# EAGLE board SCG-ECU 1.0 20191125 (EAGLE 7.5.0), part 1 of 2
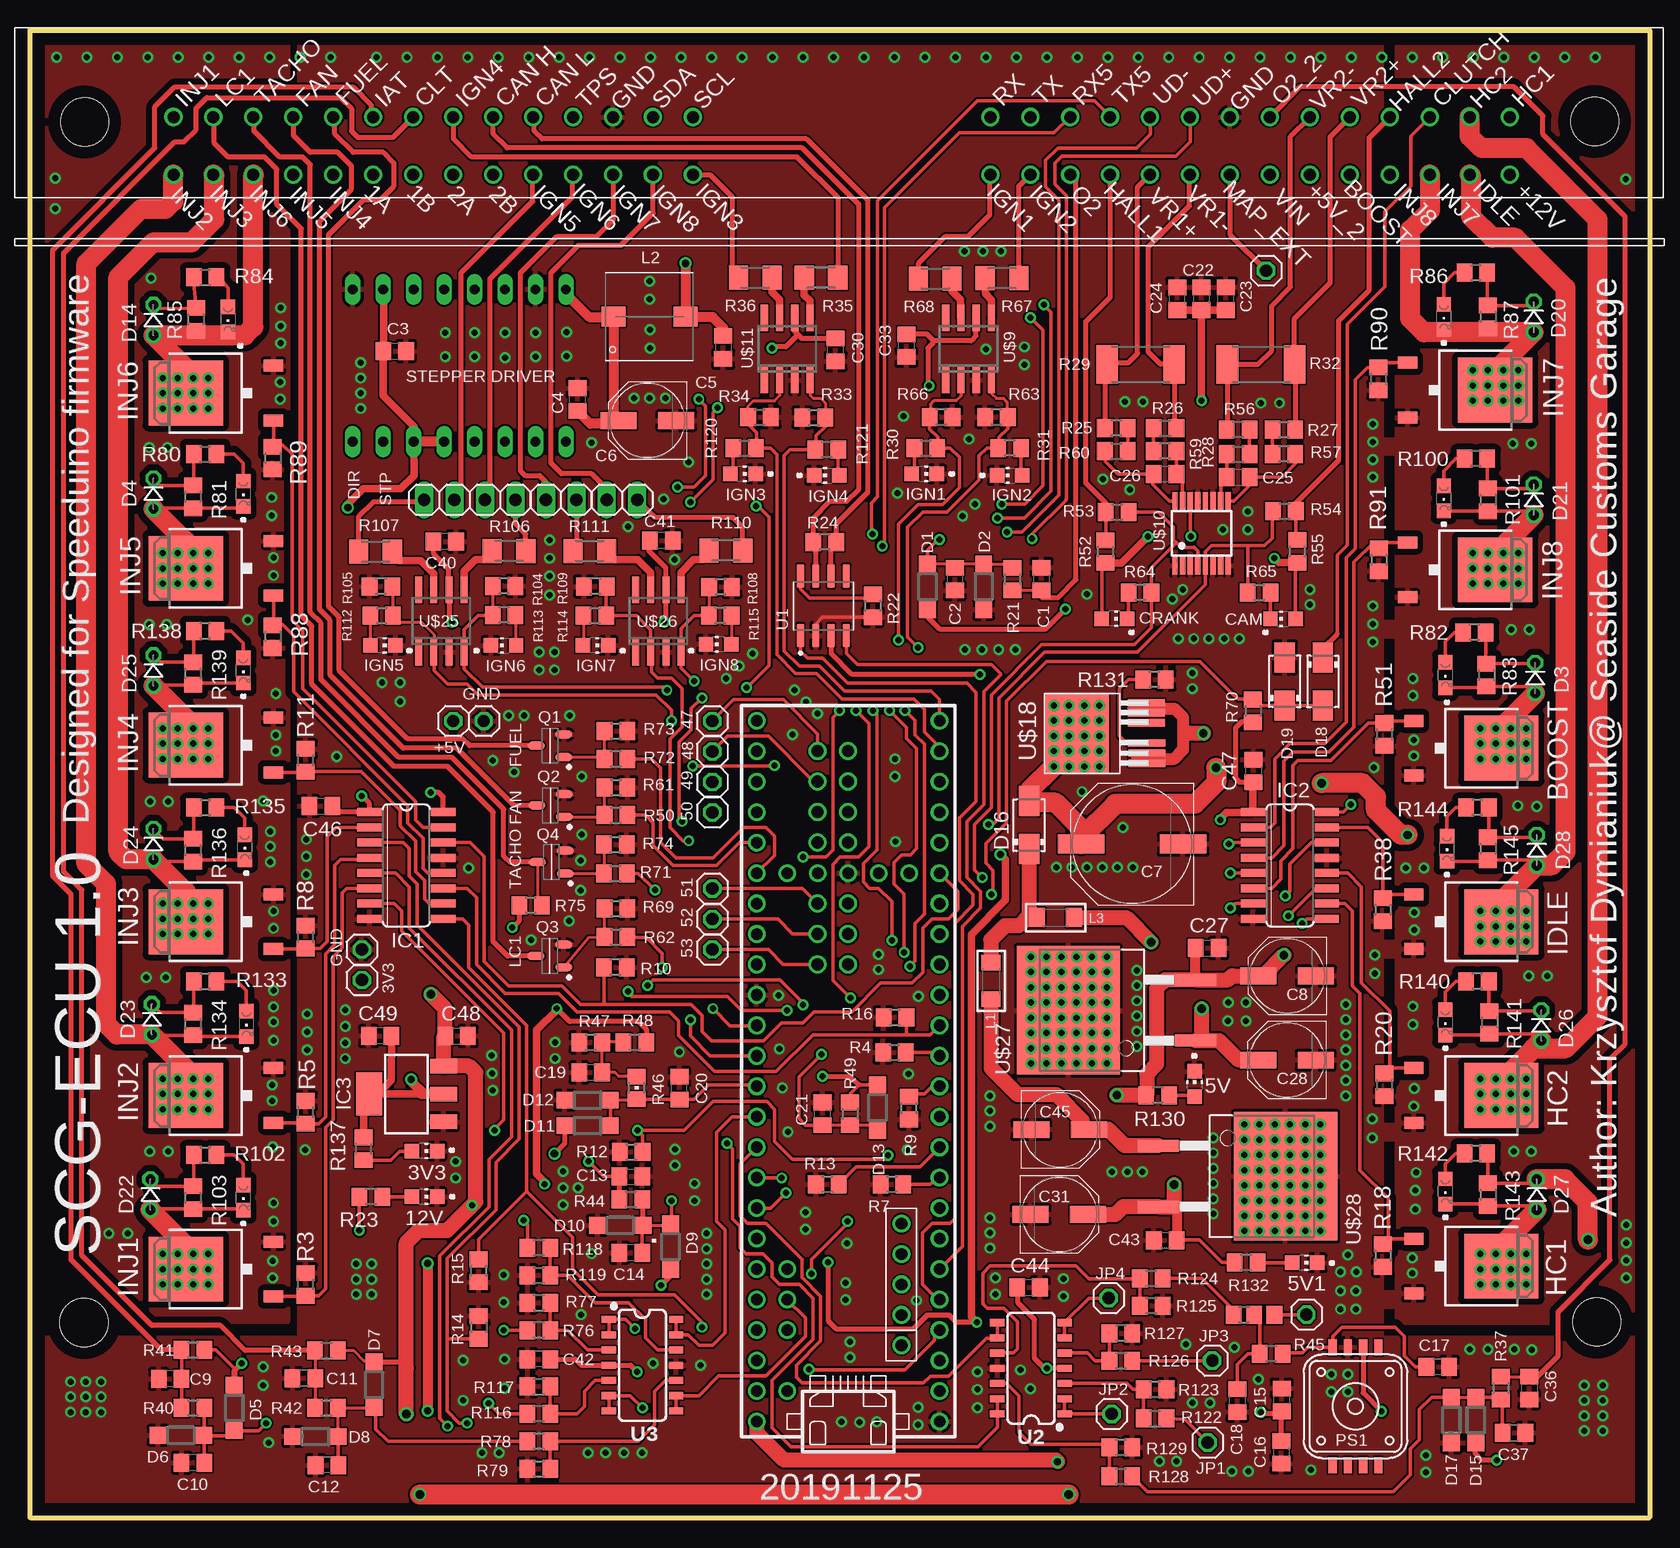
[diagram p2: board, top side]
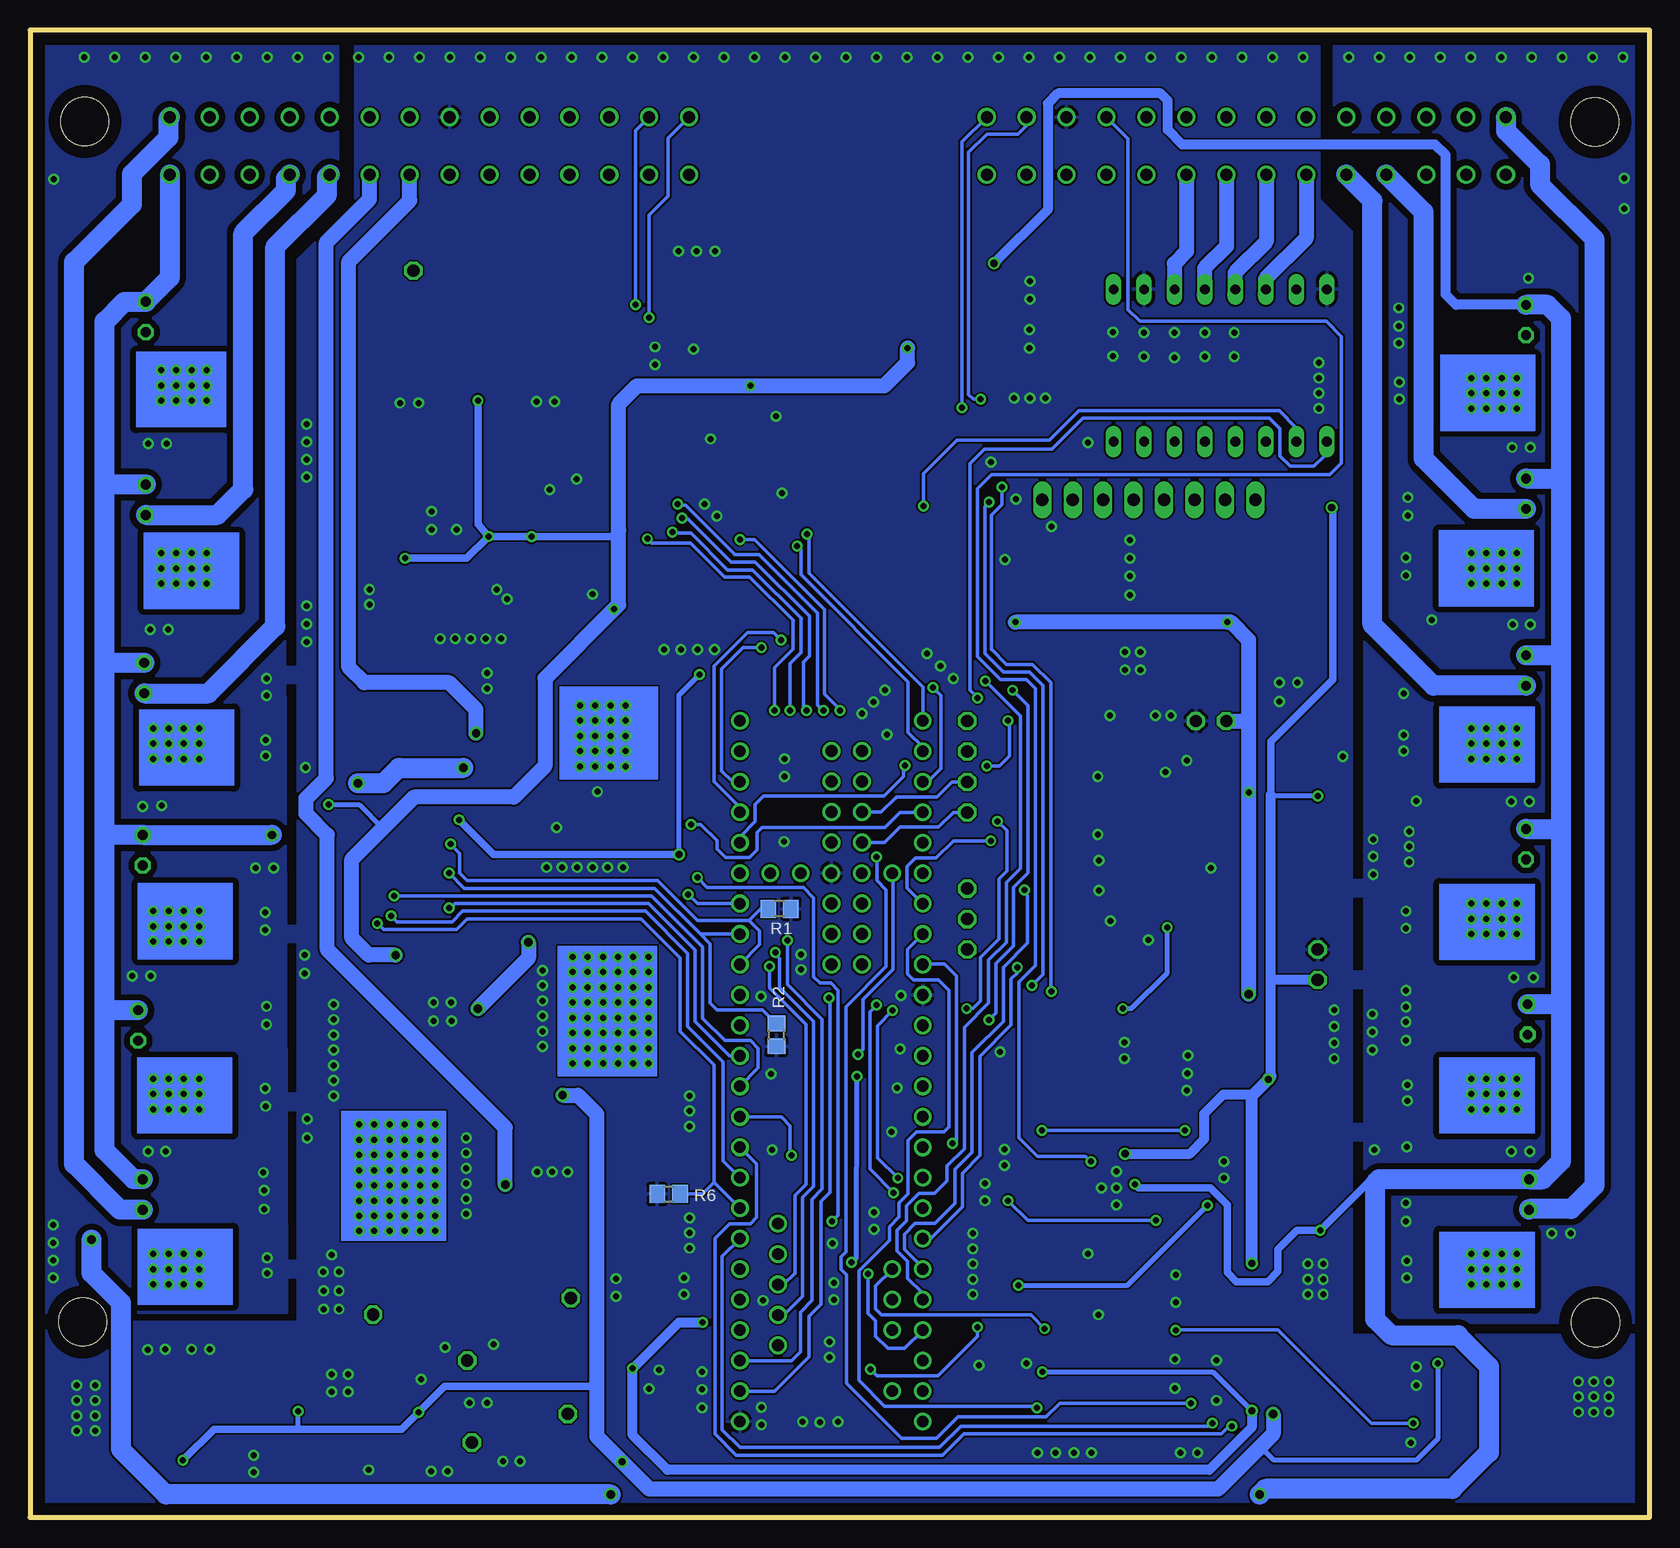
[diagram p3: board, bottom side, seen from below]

Size 135 x 124 mm. Coordinates in mm from the lower left corner, seen from the top.
Outline: 0,0 0,124 135,124 135,0 0,0
Copper layers (1*16): Top 0.035mm / dielectric 1.5mm / Bottom 0.035mm
Design rules "default *": minimum track width 10mil, minimum drill 24mil, track to track 6mil, track to pad 6mil, pad to pad 6mil, via to via 6mil, smd to smd 6mil, copper to edge 40mil, drill to drill 8mil, minimum pad ring 10mil, minimum via ring 8mil, stop-mask expansion 4mil, vias tented up to drill 20mil, thermal gap 10mil
Holes 4 mm at 4.5,16.25 130.61,16.31

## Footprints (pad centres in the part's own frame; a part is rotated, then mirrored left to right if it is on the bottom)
CHIP-LED0805 = smd 1.2 x 1.2: A 0,-1.05; C 0,1.05
C0805 = smd 1.3 x 1.5: 1 -0.95,0; 2 0.95,0
PANASONIC_D = smd 3 x 1.4: + 2.4,0; - -2.4,0
PANASONIC_G = smd 3.9 x 1.6: + 4.25,0; - -4.25,0
SOD123 = smd 1.4 x 1.4: A 1.9,0; C -1.9,0
D-2.5 = drill 0.813 octagon: A 1.27,0; C -1.27,0
DO214AC = smd 2.5 x 1.7: A 2,0; C -2,0
SO16 = smd 0.66 x 2.032: 1 -4.445,-3.073; 2 -3.175,-3.073; 3 -1.905,-3.073; 4 -0.635,-3.073; 5 0.635,-3.073; 6 1.905,-3.073; 7 3.175,-3.073; 8 4.445,-3.073; 9 4.445,3.073; 10 3.175,3.073; 11 1.905,3.073; 12 0.635,3.073; 13 -0.635,3.073; 14 -1.905,3.073; 15 -3.175,3.073; 16 -4.445,3.073
SOT223 = smd 1.219 x 2.235: 1 -2.311,-3.099; 2 0,-3.099; 3 2.311,-3.099 | smd 3.6 x 2.2: TAB 0,3.099
1X01 = drill 1.016 octagon: 1 0,0
1X02 = drill 1.016 long: 1 -1.27,0; 2 1.27,0
A0R-JMP = smd 1.5 x 1.3: 1 0,1.7; 2 0,0; 3 0,-1.7
L1206 = smd 1.3 x 1.6: 1 -1.524,0; 2 1.524,0
WE-PD_7332/7345_PLASTIC_BASE = smd 1.7 x 2: 1 0,3; 2 0,-3
CHIPLED_0805 = smd 1.2 x 1.2: A 0,-1.05; C 0,1.05
1317A = smd 1.346 x 0.686: 1 4.915,-1.905; 2 4.915,-0.635; 3 4.915,0.635; 4 4.915,1.905; 5 -4.915,1.905; 6 -4.915,0.635; 7 -4.915,-0.635; 8 -4.915,-1.905
SOT95P280X135-3N = smd 1.4 x 0.65: 1 -1.15,0.95; 2 -1.15,-0.95; 3 1.15,0
R0805 = smd 1.3 x 1.5: 1 -0.95,0; 2 0.95,0
R2512 = smd 1.8 x 3.2: 1 -2.8,0; 2 2.8,0
M1206 = smd 1.6 x 2: 1 -1.4,0; 2 1.4,0
STEP-STICK = drill 0.8 long: 1A -8.89,-7.62; 1B -8.89,-5.08; 2A -8.89,-2.54; 2B -8.89,0; DIR 3.81,-12.7; EN 3.81,5.08; GND -8.89,-12.7; GNDM -8.89,2.54; MS1 3.81,2.54; MS2 3.81,0; MS3 3.81,-2.54; RST 3.81,-5.08; SLP 3.81,-7.62; SPT 3.81,-10.16; VCC -8.89,-10.16; VMOT -8.89,5.08
SOIC127P600X175-8N = smd 1.97 x 0.6: 1 -2.475,1.905; 2 -2.475,0.635; 3 -2.475,-0.635; 4 -2.475,-1.905; 5 2.475,-1.905; 6 2.475,-0.635; 7 2.475,0.635; 8 2.475,1.905
SO14 = smd 0.6 x 1.2: 1 -3.175,-2.8; 2 -1.905,-2.8; 3 -0.635,-2.8; 4 0.635,-2.8; 5 1.905,-2.8; 6 3.175,-2.8; 7 4.445,-2.8; 8 4.445,2.8; 9 3.175,2.8; 10 1.905,2.8; 11 0.635,2.8; 12 -0.635,2.8; 13 -1.905,2.8; 14 -3.175,2.8
TEENSY_3.5/3.6 = drill 0.965: 0/RX -25.4,-7.62; 1/TX -22.86,-7.62; 2 -20.32,-7.62; 3/CANTX -17.78,-7.62; 3V3 7.62,-7.62; 3V3_2 17.78,-2.54; 3V3_LO -22.86,7.62; 4/CANRX -15.24,-7.62; 5 -12.7,-7.62; 6 -10.16,-7.62; 7 -7.62,-7.62; 8 -5.08,-7.62; 9/CS -2.54,-7.62; 10/CS 0,-7.62; 11/MOSI 2.54,-7.62; 12/MISO 5.08,-7.62; 13/SCK 5.08,7.62; 14/A0 2.54,7.62; 15/A1 0,7.62; 16/A2 -2.54,7.62; 17/A3 -5.08,7.62; 18/A4/SDA -7.62,7.62; 19/A5/SCL -10.16,7.62; 20/A6 -12.7,7.62; 21/A7 -15.24,7.62; 21/DAC0 12.7,7.62; 22/A8 -17.78,7.62; 23/A9 -20.32,7.62; 24 10.16,-7.62; 25 12.7,-7.62; 26 15.24,-7.62; 27 17.78,-7.62; 28 20.32,-7.62; 29 22.86,-7.62; 30 25.4,-7.62; 31/A12 27.94,-7.62; 32/A13 30.48,-7.62; 33/A14 30.48,7.62; 34/A15 27.94,7.62; 35/A16 25.4,7.62; 36/A17 22.86,7.62; 37/A18 20.32,7.62; 38/A19 17.78,7.62; 39/A20 15.24,7.62; A10 -17.78,5.08; A11 -15.24,5.08; A22/DAC1 10.16,7.62; AGND -25.4,7.62; AREF -20.32,5.08; GND -27.94,-7.62; GND2 7.62,7.62; GND3 17.78,0; PROG 17.78,2.54; RESET 17.78,5.08; U5V -21.59,-4.445; UD+ -16.51,-4.445; UD- -19.05,-4.445; UGND1 -13.97,-4.445; UGND2 -11.43,-4.445; VBAT 17.78,-5.08; VIN -27.94,7.62; VUSB -25.4,5.08 | drill 1: 40 10.16,0; 41 12.7,0; 42 15.24,0; 43 20.32,0; 44 22.86,0; 45 25.4,0; 46 27.94,0; 47 27.94,2.54; 48 25.4,2.54; 49 22.86,2.54; 50 20.32,2.54; 51 15.24,2.54; 52 12.7,2.54; 53 10.16,2.54
DPAK_N-CHANNEL_MOSFET = smd 5.4 x 6.2: D 0,1.23 | smd 1 x 1.6: G -2.28,-6.07; S 2.28,-6.07
SO-8 = smd 0.6 x 2.2: 1 -1.905,-2.6; 2 -0.635,-2.6; 3 0.635,-2.6; 4 1.905,-2.6; 5 1.905,2.6; 6 0.635,2.6; 7 -0.635,2.6; 8 -1.905,2.6
QSOP16 = smd 0.45 x 1.5: 1 -2.223,-2.69; 2 -1.587,-2.69; 3 -0.953,-2.69; 4 -0.318,-2.69; 5 0.318,-2.69; 6 0.953,-2.69; 7 1.587,-2.69; 8 2.223,-2.69; 9 2.223,2.69; 10 1.587,2.69; 11 0.953,2.69; 12 0.318,2.69; 13 -0.318,2.69; 14 -0.953,2.69; 15 -1.587,2.69; 16 -2.223,2.69
56PIN_CONNECTOR = drill 1: 1 -55.35,1.66; 2 -52.02,1.66; 3 -48.69,1.66; 4 -45.36,1.66; 5 -42.03,1.66; 6 -38.7,1.66; 7 -35.37,1.66; 8 -32.04,1.66; 9 -28.71,1.66; 10 -25.38,1.66; 11 -22.05,1.66; 12 -18.72,1.66; 13 -15.39,1.66; 14 -12.06,1.66; 15 -55.35,-3.14; 16 -52.02,-3.14; 17 -48.69,-3.14; 18 -45.36,-3.14; 19 -42.03,-3.14; 20 -38.7,-3.14; 21 -35.37,-3.14; 22 -32.04,-3.14; 23 -28.71,-3.14; 24 -25.38,-3.14; 25 -22.05,-3.14; 26 -18.72,-3.14; 27 -15.39,-3.14; 28 -12.06,-3.14; 29 12.74,1.66; 30 16.07,1.66; 31 19.4,1.66; 32 22.73,1.66; 33 26.06,1.66; 34 29.39,1.66; 35 32.72,1.66; 36 36.05,1.66; 37 39.38,1.66; 38 42.71,1.66; 39 46.04,1.66; 40 49.37,1.66; 41 52.7,1.66; 42 56.03,1.66; 43 12.74,-3.14; 44 16.07,-3.14; 45 19.4,-3.14; 46 22.73,-3.14; 47 26.06,-3.14; 48 29.39,-3.14; 49 32.72,-3.14; 50 36.05,-3.14; 51 39.38,-3.14; 52 42.71,-3.14; 53 46.04,-3.14; 54 49.37,-3.14; 55 52.7,-3.14; 56 56.03,-3.14 | hole 4: -62.76,1.24; 63.12,1.28
VN5R003H-E_HPAK_TO267_7 = smd 0.6 x 3.1: 1 -2.53,1.65; 2 -1.68,1.65; 3 -0.83,1.66; 5 0.85,1.67; 6 1.68,1.67; 7 2.53,1.67 | smd 6.5 x 5.3: 4 -0.05,7.45
TO263-3 = smd 1 x 3.4: 1 -2.54,-6.6; 3 2.54,-6.6 | smd 10.7 x 8.6: TAB 0,4

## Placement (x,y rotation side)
3V3  [CHIP-LED0805]  32.89,30.56 270 top
5V  [CHIP-LED0805]  97.08,36.14 0 top
5V1  [CHIP-LED0805]  106.25,21.23 270 top
12V  [CHIP-LED0805]  32.89,26.75 270 top
C1  100nF  [C0805]  84.33,78.23 90 top
C2  220nF  [C0805]  77.09,78.23 270 top
C3  100nF  [C0805]  30.4,97.23 0 top
C4  100nF 50V  [C0805]  45.64,93.19 90 top
C5  100nF 50V  [C0805]  57.78,97.54 270 top
C6  100uF 35V  [PANASONIC_D]  51.46,91.44 180 top
C7  470uF 50V  [PANASONIC_G]  91.87,56.13 180 top
C8  220uF  [PANASONIC_D]  104.8,45.14 180 top
C9  100nF  [C0805]  11.68,11.56 180 top
C10  220nF  [C0805]  13.59,4.57 180 top
C11  100nF  [C0805]  22.83,11.61 180 top
C12  220nF  [C0805]  24.77,4.37 180 top
C13  100nF  [C0805]  50.09,28.42 0 top
C14  220nF  [C0805]  50.09,22.07 180 top
C15  1uF  [C0805]  104.34,9.8 90 top
C16  100nF  [C0805]  104.29,5.44 270 top
C17  100nF  [C0805]  117.35,12.55 180 top
C18  220nF  [C0805]  100.63,9.75 90 top
C19  100nF  [C0805]  46.74,37.08 180 top
C20  220nF  [C0805]  54.13,35.79 90 top
C21  4.7nF  [C0805]  66.07,33.66 90 top
C22  10nF  [C0805]  97.66,101.6 90 top
C23  100nF  [C0805]  99.69,101.6 90 top
C24  1uF  [C0805]  95.63,101.6 90 top
C25  1nF  [C0805]  100.71,86.74 0 top
C26  1nF  [C0805]  94.61,86.99 0 top
C27  1uF  [C0805]  98.12,47.47 0 top
C28  220uF  [PANASONIC_D]  104.78,38.13 180 top
C30  1uF  [C0805]  67.16,97.33 90 top
C31  220uF  [PANASONIC_D]  85.8,25.27 0 top
C33  1uF  [C0805]  73.05,97.69 90 top
C36  100nF  [C0805]  124.97,10.79 270 top
C37  220nF  [C0805]  123.7,7.06 0 top
C40  1uF  [C0805]  34.57,81.36 180 top
C41  1uF  [C0805]  52.63,81.43 180 top
C42  100nF  [C0805]  42.42,13.21 180 top
C43  1uF  [C0805]  94.64,23.09 180 top
C44  100nF  [C0805]  83.24,19.18 0 top
C45  220uF  [PANASONIC_D]  85.88,32.33 0 top
C46  100nF  [C0805]  24.26,59.31 0 top
C47  100nF  [C0805]  101.98,62.23 270 top
C48  10uF  [C0805]  35.56,40.13 0 top
C49  10uF  [C0805]  29.18,40.13 180 top
D1  1N5819HW-7-F  [SOD123]  74.8,77.6 90 top
D2  1N5819HW-7-F  [SOD123]  79.5,77.6 270 top
D3  1N4001  [D-2.5]  125.48,69.98 270 top
D4  1N4001  [D-2.5]  10.29,85.34 270 top
D5  1N5819HW-7-F  [SOD123]  17.02,9.14 270 top
D6  1N5819HW-7-F  [SOD123]  12.57,6.86 180 top
D7  1N5819HW-7-F  [SOD123]  28.68,11.07 270 top
D8  1N5819HW-7-F  [SOD123]  23.8,6.76 180 top
D9  1N5819HW-7-F  [SOD123]  53.39,22.58 90 top
D10  1N5819HW-7-F  [SOD123]  49.2,24.36 180 top
D11  1N5819  [SOD123]  46.48,32.66 0 top
D12  1N5819  [SOD123]  46.48,34.8 180 top
D13  1N5819HW-7-F  [SOD123]  70.64,34.16 270 top
D14  1N4001  [D-2.5]  10.29,99.82 270 top
D15  1N5819HW-7-F  [SOD123]  120.52,8.13 90 top
D16  B340A 3A  [DO214AC]  83.29,57.71 90 top
D17  1N5819HW-7-F  [SOD123]  118.49,8.13 270 top
D18  1N4001 SMA  [DO214AC]  107.77,69.7 270 top
D19  1N4001 SMA  [DO214AC]  104.6,69.7 90 top
D20  1N4001  [D-2.5]  125.35,100.08 270 top
D21  1N4001  [D-2.5]  125.35,84.84 270 top
D22  1N4001  [D-2.5]  10.03,26.92 270 top
D23  1N4001  [D-2.5]  10.16,41.53 270 top
D24  1N4001  [D-2.5]  10.29,56.13 270 top
D25  1N4001  [D-2.5]  10.29,70.61 270 top
D26  1N4001  [D-2.5]  125.98,41.02 270 top
D27  1N4001  [D-2.5]  125.6,26.92 270 top
D28  1N4001  [D-2.5]  125.6,55.63 270 top
IC1  4504D  [SO16]  31.37,54.36 270 top
IC2  4504D  [SO16]  105.03,54.36 270 top
IC3  LM1117IMPX-3.3  [SOT223]  31.37,35.31 90 top
JP1  [1X01]  98.17,6.25 0 top
JP2  [1X01]  90.17,8.64 0 top
JP3  [1X01]  98.55,13.08 0 top
JP4  [1X01]  89.92,18.29 0 top
JP5  [1X01]  56.87,47.35 0 top
JP6  [1X01]  56.87,49.89 0 top
JP7  [1X01]  56.87,52.43 0 top
JP8  [1X01]  56.87,58.78 0 top
JP9  [1X01]  56.87,61.32 0 top
JP10  [1X01]  56.87,63.86 0 top
JP11  [1X01]  56.87,66.4 0 top
JP12  [1X01]  27.66,47.35 0 top
JP13  [1X01]  35.28,66.4 0 top
JP14  [1X01]  27.66,44.81 0 top
JP15  [1X02]  34.11,84.84 0 top
JP16  [1X02]  44.27,84.84 180 top
JP17  [1X02]  49.35,84.84 0 top
JP18  [1X02]  39.19,84.84 0 top
JP19  [1X01]  37.82,66.4 0 top
JP20  0R-JUMPA  [A0R-JMP]  102.03,16.92 90 top
JP21  [1X01]  106.4,16.92 0 top
JP22  [1X01]  103.05,103.94 0 top
L1  600R 2A  [L1206]  80.11,44.73 90 top
L2  8.2uH 2.7A  [WE-PD_7332/7345_PLASTIC_BASE]  51.64,100.1 90 top
L3  600R 2A  [L1206]  85.5,50.01 180 top
LED1  [CHIP-LED0805]  74.55,86.99 270 top
LED2  [CHIP-LED0805]  81.66,86.87 90 top
LED3  [CHIP-LED0805]  59.44,86.99 270 top
LED4  [CHIP-LED0805]  66.42,86.87 90 top
LED5  [CHIPLED_0805]  117.98,70.23 180 top
LED6  [CHIP-LED0805]  90.4,74.93 270 top
LED7  [CHIP-LED0805]  104.44,74.9 90 top
LED8  [CHIPLED_0805]  17.78,85.34 180 top
LED9  [CHIPLED_0805]  16.51,99.87 180 top
LED10  [CHIPLED_0805]  117.86,100.08 180 top
LED11  [CHIPLED_0805]  117.86,84.96 180 top
LED12  [CHIPLED_0805]  17.78,26.67 180 top
LED13  [CHIPLED_0805]  18.03,41.15 180 top
LED14  [CHIPLED_0805]  17.91,55.88 180 top
LED15  [CHIPLED_0805]  17.78,70.61 180 top
LED16  [CHIPLED_0805]  117.98,41.28 180 top
LED17  [CHIPLED_0805]  117.98,27.18 180 top
LED18  [CHIPLED_0805]  118.11,55.75 180 top
LED20  [CHIP-LED0805]  29.41,72.69 270 top
LED21  [CHIP-LED0805]  39.47,72.69 90 top
LED22  [CHIP-LED0805]  47.14,72.69 270 top
LED23  [CHIP-LED0805]  57.4,72.8 90 top
PS1  MPXH6400AC6T1  [1317A]  110.49,9.27 90 top
Q1  IRLML0030TRPBF  [SOT95P280X135-3N]  43.36,64.34 180 top
Q2  IRLML0030TRPBF  [SOT95P280X135-3N]  43.38,59.36 180 top
Q3  IRLML0030TRPBF  [SOT95P280X135-3N]  43.33,46.81 180 top
Q4  IRLML0030TRPBF  [SOT95P280X135-3N]  43.46,54.64 180 top
R1  10K  [R0805]  72.52,50.75 180 bottom
R2  10K  [R0805]  72.77,40.23 90 bottom
R3  68K  [R0805]  22.99,19.43 90 top
R4  10K  [R0805]  72.06,38.76 0 top
R5  68K  [R0805]  22.99,33.78 90 top
R6  10K  [R0805]  81.76,26.97 0 bottom
R7  10K  [R0805]  71.86,27.79 0 top
R8  68K  [R0805]  22.99,48.39 90 top
R9  10K  [R0805]  73.28,34.14 90 top
R10  10K  [R0805]  48.79,45.87 180 top
R11  68K  [R0805]  22.99,63.12 90 top
R12  10K  [R0805]  50.11,30.48 0 top
R13  10K  [R0805]  66.47,27.79 0 top
R14  10K  [R0805]  37.41,15.85 270 top
R15  10K  [R0805]  37.41,20.57 90 top
R16  10K  [R0805]  72.11,41.71 0 top
R18  68K  [R0805]  112.78,21.84 270 top
R20  68K  [R0805]  112.9,36.07 270 top
R21  470R  [R0805]  81.92,78.23 90 top
R22  10K  [R0805]  70.26,76 270 top
R23  2K7  [R0805]  28.42,26.75 180 top
R24  120R  [R0805]  66.24,81.31 180 top
R25  5K  [R0805]  90.55,90.8 180 top
R26  5K  [R0805]  94.61,90.8 0 top
R27  5K  [R0805]  104.52,90.68 0 top
R28  5K  [R0805]  100.71,88.65 0 top
R29  4K7 3W  [R2512]  92.58,96.14 0 top
R30  470R  [R0805]  74.68,89.15 0 top
R31  470R  [R0805]  81.66,89.15 180 top
R32  4K7 3W  [R2512]  102.62,96.14 0 top
R33  100K  [R0805]  65.33,91.69 0 top
R34  100K  [R0805]  60.81,91.72 0 top
R35  22R  [M1206]  65.94,103.35 0 top
R36  22R  [M1206]  60.45,103.35 180 top
R37  470R  [R0805]  122.61,10.79 270 top
R38  68K  [R0805]  112.78,50.67 270 top
R40  470R  [R0805]  13.59,9.14 0 top
R41  2K49  [R0805]  13.59,13.97 0 top
R42  470R  [R0805]  24.71,9.14 0 top
R43  2K49  [R0805]  24.71,13.92 0 top
R44  470R  [R0805]  50.09,26.52 0 top
R45  470R  [R0805]  103.45,13.64 180 top
R46  470R  [R0805]  50.55,35.81 270 top
R47  1K  [R0805]  46.74,39.62 0 top
R48  3K9  [R0805]  50.42,39.62 0 top
R49  1K  [R0805]  68.35,33.66 270 top
R50  100R  [R0805]  48.84,58.55 0 top
R51  68K  [R0805]  112.9,65.28 270 top
R52  10K  [R0805]  89.66,80.52 90 top
R53  1K  [R0805]  90.63,83.82 0 top
R54  1K  [R0805]  104.57,83.9 0 top
R55  10K  [R0805]  105.64,80.54 90 top
R56  5K  [R0805]  100.71,90.68 180 top
R57  5K  [R0805]  104.52,88.65 180 top
R59  5K  [R0805]  94.61,88.9 180 top
R60  5K  [R0805]  90.55,88.9 0 top
R61  47K  [R0805]  48.84,60.86 0 top
R62  100R  [R0805]  48.84,48.39 0 top
R63  100K  [R0805]  80.57,91.74 0 top
R64  10K  [R0805]  92.53,77.11 180 top
R65  10K  [R0805]  102.46,77.11 0 top
R66  100K  [R0805]  75.95,91.74 0 top
R67  22R  [M1206]  81.03,103.3 0 top
R68  22R  [M1206]  75.46,103.28 180 top
R69  47K  [R0805]  48.84,50.77 0 top
R70  2,2K  [R0805]  101.96,67.23 270 top
R71  100R  [R0805]  48.79,53.7 0 top
R72  100R  [R0805]  48.84,63.25 0 top
R73  47K  [R0805]  48.84,65.56 0 top
R74  47K  [R0805]  48.79,56.11 0 top
R75  10K  [R0805]  41.73,51.03 180 top
R76  180K +/-0.1%  [R0805]  42.42,15.62 180 top
R77  330K +/-0.1%  [R0805]  42.42,17.91 0 top
R78  180K +/-0.1%  [R0805]  42.42,6.35 180 top
R79  330K +/-0.1%  [R0805]  42.42,4.06 0 top
R80  2K7  [R0805]  14.61,88.65 0 top
R81  1K  [R0805]  13.59,85.09 270 top
R82  2K7  [R0805]  120.4,73.79 180 top
R83  1K  [R0805]  121.41,70.23 270 top
R84  2K7  [R0805]  14.61,103.38 0 top
R85  1K  [R0805]  13.84,99.87 270 top
R86  2K7  [R0805]  120.52,103.76 180 top
R87  1K  [R0805]  121.54,100.08 270 top
R88  68K  [R0805]  20.24,73.43 270 top
R89  68K  [R0805]  20.24,88.32 270 top
R90  68K  [R0805]  112.39,94.92 270 top
R91  68K  [R0805]  112.45,79.83 270 top
R100  2K7  [R0805]  120.52,88.27 180 top
R101  1K  [R0805]  121.54,84.84 270 top
R102  2K7  [R0805]  14.61,30.23 0 top
R103  1K  [R0805]  13.59,26.67 270 top
R104  100K  [R0805]  39.52,77.65 180 top
R105  100K  [R0805]  29.26,77.62 180 top
R106  22R  [M1206]  39.93,80.57 0 top
R107  22R  [M1206]  28.8,80.52 180 top
R108  100K  [R0805]  57.56,77.57 180 top
R109  100K  [R0805]  47.12,77.62 180 top
R110  22R  [M1206]  58.01,80.62 0 top
R111  22R  [M1206]  46.66,80.57 180 top
R112  470R  [R0805]  29.31,75.18 0 top
R113  470R  [R0805]  39.52,75.23 180 top
R114  470R  [R0805]  47.09,75.18 0 top
R115  470R  [R0805]  57.53,75.18 180 top
R116  180K +/-0.1%  [R0805]  42.42,8.64 180 top
R117  330K +/-0.1%  [R0805]  42.42,10.92 0 top
R118  180K +/-0.1%  [R0805]  42.42,22.48 180 top
R119  330K +/-0.1%  [R0805]  42.42,20.19 0 top
R120  470R  [R0805]  59.56,89.15 0 top
R121  470R  [R0805]  66.42,89.03 180 top
R122  180K +/-0.1%  [R0805]  93.78,8.26 0 top
R123  330K +/-0.1%  [R0805]  93.78,10.67 180 top
R124  180K +/-0.1%  [R0805]  93.47,19.94 0 top
R125  330K +/-0.1%  [R0805]  93.47,17.65 180 top
R126  180K +/-0.1%  [R0805]  90.93,13.08 0 top
R127  330K +/-0.1%  [R0805]  90.93,15.37 180 top
R128  180K +/-0.1%  [R0805]  90.93,3.43 0 top
R129  330K +/-0.1%  [R0805]  90.93,5.84 180 top
R130  560R  [R0805]  94.01,35.2 180 top
R131  100R  [R0805]  93.73,69.85 180 top
R132  560R  [R0805]  101.37,21.26 180 top
R133  2K7  [R0805]  14.61,44.7 0 top
R134  1K  [R0805]  13.59,41.15 270 top
R135  2K7  [R0805]  14.61,59.18 0 top
R136  1K  [R0805]  13.59,55.63 270 top
R137  470R  [R0805]  27.81,30.73 90 top
R138  2K7  [R0805]  14.61,73.91 0 top
R139  1K  [R0805]  13.59,70.36 270 top
R140  2K7  [R0805]  120.65,44.7 180 top
R141  1K  [R0805]  121.67,41.28 270 top
R142  2K7  [R0805]  120.52,30.35 180 top
R143  1K  [R0805]  121.54,26.92 270 top
R144  2K7  [R0805]  120.65,59.18 180 top
R145  1K  [R0805]  121.54,55.75 270 top
STEPSTICK-X  STEP-STICK  [STEP-STICK]  39.6,93.5 270 top
U1  SN65HVD230QDR  [SOIC127P600X175-8N]  66.14,76 90 top
U2  LMV324  [SO14]  83.44,11.81 90 top
U3  LMV324  [SO14]  51.05,13.34 270 top
U$1  TEENSY_3.5/3.6  [TEENSY_3.5/3.6]  68.2,35.94 90 top
U$2  DPAK_N-CHANNEL_MOSFET  [DPAK_N-CHANNEL_MOSFET]  121.41,35.18 270 top
U$3  DPAK_N-CHANNEL_MOSFET  [DPAK_N-CHANNEL_MOSFET]  121.41,20.95 270 top
U$4  DPAK_N-CHANNEL_MOSFET  [DPAK_N-CHANNEL_MOSFET]  14.22,35.18 90 top
U$5  DPAK_N-CHANNEL_MOSFET  [DPAK_N-CHANNEL_MOSFET]  121.41,49.66 270 top
U$6  DPAK_N-CHANNEL_MOSFET  [DPAK_N-CHANNEL_MOSFET]  14.22,49.66 90 top
U$8  DPAK_N-CHANNEL_MOSFET  [DPAK_N-CHANNEL_MOSFET]  14.22,64.39 90 top
U$9  TC427SO-8  [SO-8]  78.23,97.41 0 top
U$10  MAX9926  [QSOP16]  97.66,82.04 0 top
U$11  TC427SO-8  [SO-8]  63.12,97.41 0 top
U$12  DPAK_N-CHANNEL_MOSFET  [DPAK_N-CHANNEL_MOSFET]  14.22,20.7 90 top
U$13  DPAK_N-CHANNEL_MOSFET  [DPAK_N-CHANNEL_MOSFET]  121.41,64.13 270 top
U$17  56PIN_CONNECTOR  [56PIN_CONNECTOR]  67.31,115.09 0 top
U$18  VN5R003H-E  [VN5R003H-E_HPAK_TO267_7]  94.74,65.41 90 top
U$19  DPAK_N-CHANNEL_MOSFET  [DPAK_N-CHANNEL_MOSFET]  14.22,79.12 90 top
U$20  DPAK_N-CHANNEL_MOSFET  [DPAK_N-CHANNEL_MOSFET]  14.22,93.73 90 top
U$21  DPAK_N-CHANNEL_MOSFET  [DPAK_N-CHANNEL_MOSFET]  120.9,93.98 270 top
U$22  DPAK_N-CHANNEL_MOSFET  [DPAK_N-CHANNEL_MOSFET]  120.9,78.99 270 top
U$25  TC427SO-8  [SO-8]  34.29,74.73 0 top
U$26  TC427SO-8  [SO-8]  52.37,74.73 0 top
U$27  MIC29301-5.0WU-TR  [TO263-3]  90.55,42.29 90 top
U$28  MIC29301-5.0WU-TR  [TO263-3]  100.66,28.45 270 top

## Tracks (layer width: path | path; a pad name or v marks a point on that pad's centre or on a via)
+3V3  (via drill 0.5, 0.6)
  Top 0.305: D13.C 69.11,36.06 68.4,35.36 68.4,34.66 R49.1
  Top 0.406: C46.2 25.71,58.8 IC1.1 28.3,59.51 v27.66,60.15 | 101.96,61.26 C47.2 100.85,61.28 100.51,61.62 100.51,65.84 101.02,66.34 101.89,66.34 R70.2 | C42.1 45.47,13.21 45.97,12.7 U3.4 50.06,12.7 v50.62,12.14 | U2.4 v84.76,12.45 84.56,12.45 83.74,13.26 83.74,16.51 82.37,17.88 82.37,19.09 C44.1 | D11.C 44.58,31.2 v43.71,30.33 | v78.92,16.26 77.24,16.26 76.63,16.87 74.75,16.87 73.58,15.7 67.23,15.7 66.57,16.36 66.57,21.23 v66.52,21.29 | v99.24,58.17 99.24,58.27 | 101.93,58.78 IC2.1 | U1.3 66.8,73.5 66.8,72.01 68.53,70.28 v79.2,70.28 | D13.C | v66.06,36.78 68.34,36.78 69.11,36.06
  Top 0.61: IC2.1 101.96,61.26 | R137.2 27.81,35.05 27.56,35.31 | 27.56,35.31 IC3.TAB 28.98,35.31 | 27.69,35.43 27.56,35.31 | 28.98,35.31 32.64,35.31 32.84,35.31 IC3.2 | C49.1 30.11,36.44 28.98,35.31 | C3.1 29.45,93.51 32.03,90.93 STEPSTICK-X.SLP 32.03,86.87 30.91,85.75 27.76,85.75 26.49,84.48 v26.49,84.18 | v80.9,55.27 81.31,54.86 81.31,51.46 78.46,48.62 78.46,16.71 v78.92,16.26 | 99.24,58.27 99.75,58.78 101.93,58.78 | 29.49,97.27 29.49,102.34 STEPSTICK-X.VCC
  Top 0.813: 29.49,97.27 C3.1 | STEPSTICK-X.RST STEPSTICK-X.SLP | v31.77,36.53 31.77,36.37 32.84,35.31 | IC3.2 32.64,35.31 | v33.15,21.18 v33.15,8.89
  Bottom 0.406: v50.62,12.14 36.4,12.14 v33.15,8.89 | v27.66,60.15 31.47,60.15 31.57,60.25 | v80.9,55.27 80.9,68.58 v79.2,70.28 | v66.52,21.29 66.47,21.29 66.12,21.64 v66.06,36.78
  Bottom 0.61: v80.9,55.27 96.34,55.27 v99.24,58.17 | 31.57,60.25 31.57,64.67 26.39,69.85 26.39,84.07 v26.49,84.18
  Bottom 0.813: v43.71,30.33 38.33,30.33 37.11,31.55 37.11,33.68 35.53,35.26 33.05,35.26 v31.77,36.53 | v78.92,16.26 80.9,16.26 84.71,12.45 v84.76,12.45 84.76,6.86 81.86,3.96 36.7,3.96 33.15,7.52 v33.15,8.89 | 31.57,36.78 31.57,44.81 | 31.57,44.81 31.57,60.25 | JP14.1 31.57,44.81
  Bottom 1.016: v33.15,21.18 33.15,35.15 v31.77,36.53 31.77,36.58 31.57,36.78
+5V  (via drill 0.5, 0.6, 0.7)
  Top 0.254: R43.2 26.98,13.92 27.81,13.08 28.57,13.08 D7.C
  Top 0.305: U$10.14 96.71,81.85 v96.77,81.79 | 34.9,77.35 U$25.6 | LED6.A 89.35,79.25 R52.1 | LED7.A 105.5,79.45 R55.1 | R41.2 15.49,13.97 17.14,12.32 17.14,11.17 D5.C | IC2.16 109.47,58.8 v110.11,59.44
  Top 0.406: C16.1 104.29,8.8 C15.1 103.98,8.85 103.76,8.64 102.74,8.64 v102.62,8.76 | v122.25,4.78 121.03,4.78 120.47,5.33 120.47,6.18 D15.C | C30.2 64.35,98.28 64.03,98.6 | 64.03,98.6 63.78,98.86 | 63.78,98.86 63.78,99.98 U$11.6 63.75,98.88 63.78,98.86 | 64.03,98.6 63.02,97.59 61.95,97.59 v61.85,97.48 | U$9.6 78.87,98.5 78.46,98.09 75.31,98.09 | D1.C 74.8,75.08 75.82,74.07 84.66,74.07 v86.31,75.72 | D9.C 53.39,20.14 v52.6,19.36 | IC1.16 34.44,60.07 34.06,60.45 v33.4,60.45 | v52.86,74.62 53.01,74.78 U$26.6 53.01,79.15 51.59,80.57 51.59,81.34 C41.2 | U$25.6 34.92,74.88 v35.18,74.62 | D5.C 17.02,12.22 v17.65,12.85 | D7.C 30.84,12.97 31.37,12.45 | 75.31,98.09 74.75,98.65 73.07,98.65 C33.2 | 75.31,98.09 75.31,97.94 74.85,97.48 74.85,94.44 v74.95,94.34 | PS1.2 111.12,10.38 v112.65,8.85 | 34.9,77.35 34.9,79.07 33.66,80.31 33.66,81.32 C40.2
  Top 0.61: C24.1 C22.1 | C22.1 C23.1 | C22.1 v97.66,93.12 | C30.2 67.17,98.28 67.46,97.99 | R55.1 104.1,79.59 v103.73,79.96 | R52.1 91,79.57 v93.19,81.76
  Top 0.813: U$27.3 97.15,47.45 C27.1
  Top 1.27: 102.38,45.16 100.2,45.16 99.87,44.83 U$27.3 94.64,44.83 93.9,44.09 93.9,37.8 93.09,36.98 93.09,35.24 R130.2 v90.6,35.2 | 102.38,45.16 C8.+ | v31.37,8.64 31.37,12.45 31.37,22.91 32.38,23.93 34.77,23.93 v36.85,26.01 37.16,26.31 37.16,37.08 36.6,37.64 34.49,37.64 IC3.3 34.47,39.99 C48.1 34.61,42.43 v33.4,43.64 | 102.38,45.16 102.79,45.16 v104.52,46.89 | U$1.VIN 60.58,7.06 62.87,4.78 85.52,4.78 v85.65,4.65
  Bottom 0.406: v112.65,8.85 112.7,8.8 112.7,7.42 112.65,7.37 | v110.11,59.44 107.57,59.44 105.59,57.46 | 84.45,94.39 84.4,94.34 | v52.6,19.36 43.51,19.36 v36.85,26.01 | v17.65,12.85 17.65,6.55 19.43,4.78 31.32,4.78 32.44,5.89
  Bottom 0.61: v97.66,93.12 97.66,82.8 v96.77,81.79 | v103.73,79.96 98.6,79.96 v96.77,81.79 | v96.77,81.79 96.75,81.76 v93.19,81.76 86.46,81.76 85.93,82.3 | v122.25,4.78 119.66,7.37 112.65,7.37 104.01,7.37 v102.62,8.76 100.46,10.92 88.01,10.92 87.76,11.18
  Bottom 1.27: v90.6,35.2 89.33,35.2 87.76,33.63 87.76,11.18 87.76,6.76 v85.65,4.65 83.39,2.39 35.94,2.39 32.44,5.89 31.37,6.96 v31.37,8.64 | v33.4,43.64 v33.4,60.45 33.4,66.4 | v104.52,46.89 106.76,46.89 108.18,48.31 108.18,54.86 105.59,57.46 103,60.05 94.67,60.05 92.08,62.64 92.08,69.95 v86.31,75.72 85.93,76.1 85.93,82.3 85.93,92.81 84.4,94.34 v74.95,94.34 63.78,94.34 61.85,96.27 v61.85,97.48 | 33.4,66.4 33.4,73.15 34.87,74.62 v35.18,74.62 v52.86,74.62 | JP13.1 33.4,66.4
+5V_2  (via drill 0.7)
  Top 0.305: R132.2 99.36,21.26 97.46,23.16 95.67,23.16 C43.1
  Top 0.813: U$28.3 95.59,25.91 C43.1
  Top 1.27: C31.+ 88.23,25.25 90.45,25.25 91.11,25.91 U$28.3 95.38,25.91 v95.38,27.74
  Bottom 1.27: v95.38,27.74 95.38,32.51 110.21,47.35 110.21,56.9 111.99,58.67 111.99,59.94 110.31,61.62 110.31,106.27 106.7,109.88 106.7,111.93 U$17.51
+12V  (via drill 0.5, 0.6, 0.7)
  Top 0.305: R84.1 13.59,103.31 R85.1 10.61,100.77 D14.C | R80.1 13.65,86.11 R81.1 10.86,86.04 D4.C | R138.1 13.65,71.37 R139.1 10.86,71.31 D25.C | R135.1 13.65,56.64 R136.1 11.12,56.58 D24.C | R133.1 13.65,42.16 R134.1 10.86,42.1 D23.C | R102.1 13.65,27.69 R103.1 10.61,27.62 D22.C | R86.1 121.47,101.09 R87.1 125.03,101.03 D20.C | R100.1 121.47,85.85 R101.1 125.03,85.79 D21.C | R82.1 121.35,71.25 R83.1 125.41,71.18 D3.C | D28.C 125.41,56.7 R145.1 121.6,56.76 R144.1 | R140.1 121.6,42.29 R141.1 125.92,42.23 D26.C | R142.1 121.54,30.29 R143.1 125.28,27.87 D27.C | v27.46,23.93 27.46,26.73 R23.2
  Top 0.406: R48.2 51.44,39.69 51.44,40.64 50.72,41.35 44.98,41.35 v43.92,42.42 43.97,42.37 | R75.2 40.78,49.75 v40.21,49.17
  Top 0.61: v42.9,27.79 42.9,27.99 42.24,28.65 42.24,40.64 43.97,42.37
  Top 0.813: C5.1 57.78,99.19 56.9,100.08 54.66,100.08 L2.2 v54.63,104.55
  Top 1.676: U$18.4 85.98,64.04 85.98,63.25 v85.34,62.61 83.29,60.55 D16.A 83.41,59.59 85.47,59.59 87.62,57.44 87.62,56.64 | C7.+ 87.62,56.64 | v114.83,56.9 114.28,56.9 112.19,58.98 112.19,60.1 111.07,61.21 v107.67,61.21 | v98.88,62.48 98.88,61.27 97.1,59.49 90.47,59.49 87.62,56.64 | v32.49,1.93 v86.59,1.93 | v129.87,23.16 129.87,26.26 127.94,28.19 D27.C
  Bottom 0.305: D22.C 23.19,28.19
  Bottom 0.406: v43.92,42.42 43.2,42.42 40.21,45.41 v40.21,49.17
  Bottom 0.61: 23.19,28.19 v27.46,23.93 29.39,23.93 30.96,22.35 30.96,20.52 31.83,19.66 34.42,19.66 35.18,20.42 35.18,26.06 36.6,27.48 42.6,27.48 v42.9,27.79
  Bottom 0.813: D14.C 16.13,101.09 16.99,101.96 16.99,113.59 17.86,114.45 38.94,114.45 40.16,115.67 40.16,118.11 40.77,118.72 49.3,118.72 50.16,117.86 50.16,109.02 v54.63,104.55
  Bottom 1.676: 7.37,42.8 7.37,29.72 8.89,28.19 D22.C 22.53,28.19 22.88,27.84 22.88,16.56 21.51,15.19 15.98,15.19 13.39,12.6 13.39,5.44 16.43,2.39 32.03,2.39 v32.49,1.93 | 7.37,42.8 7.37,57.4 | 7.37,57.4 7.37,71.88 | 7.37,71.88 7.37,86.74 | 7.37,86.74 7.37,99.95 8.51,101.09 D14.C | D4.C 7.49,86.61 7.37,86.74 | D25.C 7.37,71.88 | D24.C 7.37,57.4 | D23.C 7.37,42.8 | D27.C 126.36,28.19 128.78,30.61 128.78,42.42 | 128.78,42.42 128.78,56.9 | 128.78,56.9 128.78,71.12 | 128.78,71.12 128.78,85.98 | 128.78,85.98 128.78,99.69 127.13,101.35 D20.C 123.34,103.35 U$17.56 | D21.C 128.65,86.11 128.78,85.98 | D3.C 128.65,71.25 128.78,71.12 | 128.78,56.9 D28.C v114.83,56.9 | D26.C 128.65,42.29 128.78,42.42 | v107.67,61.21 105.54,61.21 104.27,62.48 v98.88,62.48 | v86.59,1.93 123.67,1.93 127.43,5.69 127.43,17.93 129.87,20.37 v129.87,23.16
A23
  Bottom 0.305: U$1.49 64.06,58.8 62.87,60 62.81,60 62.76,60.05 59.41,60.05 58.14,61.32 JP9.1
A24
  Bottom 0.305: U$1.50 63.75,56.26 62.46,57.56 59.26,57.56 58.04,58.78 JP8.1
BOOST
  Top 0.305: LED5.C 121.31,69.18 R83.2 124.9,69.28 D3.A
  Top 1.676: 122.43,64.13 U$13.D 122.01,63.5 121.79,63.5 122.43,64.13 | 122.43,64.13 122.43,65.66 D3.A
  Bottom 1.676: D3.A 120.14,68.71 114.55,74.3 114.55,105.92 110.24,110.24 110.24,111.73 U$17.52
BOOST_CPU  (via drill 0.5)
  Top 0.305: IC2.7 100.46,51.18 v100.08,50.8 | R4.2 75.34,38.76 U$1.11/MOSI
  Bottom 0.305: v100.08,50.8 99.95,50.8 99.57,51.18 83.44,51.18 79.58,47.32 79.58,41.35 76.71,38.48 U$1.11/MOSI
BOOST_TC4
  Top 0.305: U$13.G 113.09,66.41 R51.1 111.57,66.23 108.43,63.09 105.69,63.09 105.28,62.69 105.28,55.75 104.27,54.74 104.27,53.21 103.5,52.45 IC2.6
BRV_CPU
  Top 0.254: D12.C 50.48,34.8
  Top 0.305: U$1.15/A1 60.45,36.07 56.57,36.07 55.35,34.85 54.14,34.85 C20.1 50.57,34.84 R46.2 | D12.C D11.A
  Top 0.406: 50.48,34.8 R46.2
CAM_CPU  (via drill 0.5)
  Top 0.305: 101.4,81 98.48,81 97.98,80.5 U$10.5 97.98,77.79 92.33,72.14 84.58,72.14 80.77,68.33 80.77,58.29 80.26,57.79 v79.88,57.79 | 101.4,81 102.89,81 103.56,81.66 103.56,83.33 R54.1 | R65.1 101.51,80.88 101.4,81
  Bottom 0.305: v79.88,57.79 79.1,57.79 77.75,56.44 77.75,55.73 77.04,55.02 75.01,55.02 74.4,55.63 74.4,57.1 73.99,57.51 63.73,57.51 62.46,58.78 60.6,58.78 U$1.36/A17
CAN_H
  Top 0.254: U1.7 65.53,78.5 | 65.53,80.64 65.29,80.88 R24.2
  Top 0.406: U$17.9 38.61,115.32 39.75,114.17 64.36,114.17 69.09,109.45 69.09,85.72 68.07,84.71 66.67,84.71 65.29,83.33 R24.2 65.53,81.07 65.53,78.5
CAN_L
  Top 0.305: 66.78,80.89 R24.1
  Top 0.406: U1.6 66.78,80.89 | U$17.10 42.04,116.64 42.04,115.57 42.67,114.93 64.72,114.93 69.85,109.8 69.85,85.47 67.19,82.81 R24.1
CANRX
  Top 0.305: U$1.4/CANRX 77.72,22.61 77.72,49.28 79.25,50.8 79.25,52.2 78.11,53.34 78.11,58.04 78.3,58.23 79.5,59.44 79.5,68.83 80.9,70.23 80.9,70.36 80.14,71.12 68.96,71.12 68.05,72.03 U1.4
CANTX
  Top 0.305: U$1.3/CANTX 75.69,18.16 74.4,19.46 74.4,23.72 75.18,24.51 76.71,24.51 77.09,24.89 77.09,49.53 78.61,51.05 78.61,51.94 77.47,53.09 77.47,58.29 78.87,59.69 78.87,68.78 78.11,69.55 68.15,69.55 66.06,71.63 64.8,71.63 64.24,72.19 U1.1
CLT
  Top 0.254: D8.C 25.66,6.79 R42.2 28.65,9.14 D7.A
  Top 0.305: D8.C 25.7,4.38 C12.1 | R78.2 29.84,6.35 28.83,7.37 28.83,9.02 D7.A
CLT_CPU
  Top 0.305: U3.8 U3.9 55.75,10.16 57.4,11.81 61.34,11.81 64.64,15.11 64.64,16.64 U$1.A10
CLUTCH_CPU  (via drill 0.5)
  Top 0.305: D18.A D19.C 102.44,67.7 R70.1 101.92,68.22 100.71,68.22 100.36,68.58 100.33,68.58 97.54,71.37 84.71,71.37 81.41,68.07 81.41,57.91 79.68,56.19 79.68,54.56 80.29,53.95 80.29,52.09 v80.14,51.94
  Bottom 0.305: U$1.26 79.38,51.18 v80.14,51.94
CLUTCH_IN
  Top 0.305: 108.97,73.66 108.97,80.24 109.8,81.08 109.8,99.47 112.95,102.62 112.95,108.86 115.09,111 115.09,115.16 U$17.40
  Top 0.406: D18.C 107.77,72.47 108.97,73.66 | 116.71,116.71 U$17.40
COOLANT_SENSOR
  Top 0.254: R43.1 23.76,11.63 C11.1 23.79,9.16 R42.1
  Top 0.406: R43.1 17.96,13.92 15.88,16 10.16,16 4.32,21.84 4.32,52.32 2.79,53.85 2.79,105.41 12.06,114.68 12.83,114.68 13.84,115.7 13.84,117.47 14.73,118.36 25.91,118.36 26.8,117.47 26.8,115.57 27.3,115.06 30.25,115.06 U$17.7
CRANK_CPU  (via drill 0.5)
  Top 0.305: U$10.4 97.35,80.58 97.03,80.9 97,80.87 95.94,80.87 95.54,81.27 | R53.2 94.08,83.82 95.33,82.57 95.33,81.48 95.54,81.27 | 95.54,81.27 93.48,79.21 R64.1 93.48,74.18 92.08,72.77 84.33,72.77 80.14,68.58 80.14,59.18 78.74,57.79 78.74,53.98 v79.38,53.34 | v65.13,20.32 65.13,21.51 68.15,24.54 v68.15,24.69
  Bottom 0.305: 79.25,53.34 v79.38,53.34 78.56,52.53 70.54,52.53 69.67,51.66 69.67,45.06 69.16,44.55 68.25,44.55 67.64,43.94 67.64,25.2 v68.15,24.69 | U$1.23/A9 62.1,14.1 63.5,14.1 64.52,15.11 64.52,16.38 65.15,17.02 65.15,20.24 v65.13,20.32
D47
  Top 0.305: JP11.1 58.65,68.17 62.81,68.17 65.66,65.33 U$1.47
D48
  Top 0.305: JP10.1 58.14,65.13 61.54,65.13 65.15,61.52 65.48,61.52 U$1.48
DIR  (via drill 0.5)
  Top 0.305: v56.01,68.33 55.12,67.44 55.12,65.66 54.1,64.64 54.1,58.29 v54.36,58.04 | v56.92,42.42 58.34,41 60.55,41 U$1.13/SCK
  Bottom 0.305: v56.01,68.33 56.64,68.96 56.64,87.86 55.45,89.05 49.81,89.05 47.22,91.64 31.67,91.64 30.81,90.78 30.81,88.49 29.95,87.63 27.96,87.63 27.1,88.49 27.1,89.48 STEPSTICK-X.DIR | v54.36,58.04 53.57,57.25 53.57,53.9 54.23,53.24 54.23,48.21 55.75,46.69 55.75,43.08 56.41,42.42 v56.92,42.42
FAN
  Top 0.406: Q2.3 40.34,59.36 35.56,64.13 31.11,64.13 25.02,70.23 25.02,74.8 24.13,75.69 24.13,108.08 26.8,110.74 26.8,112.65 25.65,113.79 23.37,113.79 21.97,115.19 21.97,116.73 U$17.4
FAN_CPU
  Top 0.305: R50.2 51.31,58.55 51.94,57.91 51.94,56.01 53.59,54.36 57.23,54.36 59.16,56.29 60.55,56.29 U$1.37/A18
FUEL
  Top 0.406: Q1.3 36.63,64.34 36.07,64.9 31.5,64.9 25.78,70.61 25.78,75.06 24.89,75.95 24.89,106.93 27.81,109.85 29.21,109.85 30.35,111 30.35,112.9 29.46,113.79 26.92,113.79 25.4,115.32 25.4,116.63 U$17.5
FUEL_CPU
  Top 0.305: R72.2 51.82,63.25 52.58,62.48 52.58,56.26 53.85,54.99 56.95,54.99 59.46,57.51 61.34,57.51 62.05,56.79 62.05,55.19 U$1.38/A19
GND  (via drill 0.5)
  Top 0.305: R22.2 66.08,75.05 65.51,74.47 U1.2
  other vias: 27.56,92.46 27.56,93.73 27.56,95 37.06,98.76 34.62,96.77 37.06,96.77 34.62,98.76 27.56,96.27 20.85,94.64 20.85,93.22 20.14,85.04 20.14,83.52 20.29,80.01 20.29,78.54 20.5,65.23 20.5,63.91 25.58,63.45 20.04,57.2 20.04,55.93 20.04,54.66 19.43,59.74 23.09,41.96 23.04,56.54 20.29,50.55 20.29,49.12 20.29,42.57 20.29,43.94 20.29,39.78 20.29,41.3 26.29,40.94 26.29,42.32 26.29,39.57 26.29,38.25 36.55,54.15 38.48,38.51 38.53,37.03 38.58,35.61 35.48,29.67 35.48,28.3 20.19,36.07 20.19,34.75 20.29,26.21 20.29,24.69 20.24,21.39 20.24,19.96 19.43,12.55 19.43,11.02 19.89,6.25 3.38,11.33 4.65,11.33 5.92,11.33 5.92,10.06 4.65,10.06 3.38,10.06 3.38,8.79 4.65,8.79 5.92,8.79 8.15,23.67 6.58,23.67 11.51,30.53 9.98,30.53 11.3,45.01 9.68,45.01 11.51,59.69 10.03,59.69 11.4,74.42 9.93,74.42 11.46,89.2 9.93,89.2 10.08,103.33 2.21,121.72 4.75,121.72 7.29,121.72 9.83,121.72 12.37,121.72 14.91,121.72 17.45,121.72 19.99,121.72 22.53,121.72 25.07,121.72 28.88,121.72 31.42,121.72 33.96,121.72 36.5,121.72 39.04,121.72 41.58,121.72 44.12,121.72 46.66,121.72 49.2,121.72 51.74,121.72 54.28,121.72 56.82,121.72 59.36,121.72 61.9,121.72 64.44,121.72 66.98,121.72 69.52,121.72 72.06,121.72 74.6,121.72 77.14,121.72 79.68,121.72 82.22,121.72 84.76,121.72 87.3,121.72 89.84,121.72 92.38,121.72 94.92,121.72 97.46,121.72 100,121.72 102.54,121.72 105.08,121.72 107.62,121.72 110.16,121.72 112.7,121.72 115.24,121.72 117.78,121.72 120.32,121.72 122.86,121.72 125.4,121.72 127.94,121.72 130.48,121.72 123.62,89.51 125.15,89.51 111.94,91.14 111.94,89.66 111.94,88.19 111.94,86.72 123.47,74.02 124.99,74.02 111.94,76 111.94,74.47 111.94,73 115.34,63.5 115.34,64.82 124.03,59.33 125.6,59.28 112.04,62.53 116.2,54.15 114.68,54.15 115.39,48.97 115.39,50.44 126.47,45.16 124.94,45.16 112.09,46.89 112.09,45.36 115.29,42.62 115.29,41.1 115.39,35.76 115.34,34.29 123.67,30.53 125.15,30.53 41.17,66.85 44.98,66.85 40.36,62.13 39.9,66.85 42.44,70.66 43.71,70.66 45.9,52.27 41.78,48.16 45.9,54.76 44.93,49.73 53.77,30.68 53.77,29.36 55.4,27.84 56.41,23.67 56.41,22.4 56.41,21.13 56.41,19.86 44.42,26.06 45.69,27.48 27.2,21.13 27.2,19.86 27.2,18.59 28.47,18.59 28.47,19.86 28.47,21.13 46.81,22 45.95,16.92 55.91,12.7 51.94,12.85 68.1,22.86 56.41,18.59 68,19.56 68,18.14 68.35,13.36 83.39,10.72 67.64,7.98 69.16,7.92 70.59,7.98 82.58,12.29 80.04,35.15 80.04,33.88 80.04,32.61 80.04,23.72 80.04,22.45 90.2,28.8 91.47,28.8 92.74,28.8 109.86,21.89 109.25,20.47 109.25,17.37 110.52,17.37 123.72,14.02 121.54,14.02 125.2,13.97 120.02,14.02 129.57,11.02 129.57,9.75 129.57,8.48 129.57,7.21 131.09,7.21 131.09,8.48 109.7,42.77 109.7,41.5 109.7,40.23 109.7,38.96 109.7,37.69 109.7,36.42 109.7,35.15 97,73.25 95.73,73.25 98.27,73.25 99.54,73.25 100.81,73.25 70.74,46.94 73.23,36.98 82.14,72.36 77.95,72.36 79.35,72.36 80.75,72.36 39.6,98.76 39.6,96.67 42.14,98.76 44.73,96.82 44.73,98.81 42.14,96.77 85.57,54.2 86.84,54.2 88.11,54.2 89.38,54.2 90.65,54.2 91.92,54.2 96.9,70.41 96.9,69.09 73.13,30.63 73.89,18.08 80.49,18.59 80.49,19.96 86.13,19.91 86.13,18.44 36.09,9.75 36.09,13.11 39.5,20.22 39.5,17.93 39.55,10.77 39.55,13.21 74.07,43.43 116.36,5.18 116.36,3.78 131.09,11.02 131.09,9.75 95.22,76.56 96.09,77.37 70.71,45.67 54.13,38.81 50.37,93.32 51.64,93.32 52.96,93.32 46.81,89.61 54.89,87.99 2.11,111.66 2.11,109.12 133.02,111.56 133.07,19.96 133.07,21.44 133.07,22.91 133.07,24.38 29.34,69.6 30.86,69.6 30.86,68.02 43.31,81.48 43.31,79.96 43.31,78.49 43.31,76.91 43.71,72.14 42.44,72.14 58.04,69.95 59.11,70.97 60.22,72.03 43.76,39.62 43.76,38.25 44.42,28.85 44.42,27.48 37.67,5.38 39.09,5.38 46.51,5.38 47.98,5.38 49.5,5.38 51.03,5.38 22.94,30.63 20.24,30.89 20.5,68.68 18.16,74.83 51.64,101.55 51.64,103.07 51.69,99.01 51.69,97.49 82.88,96.11 82.88,97.59 79.68,97.38 72.82,91.8 78.26,89.92 72.31,85.39 78.77,84.48 77.75,83.46 101.52,82.35 101.52,83.87 106.71,77.37 106.71,76.1 99.9,42.93 101.37,42.93 101.37,41.4 99.85,41.4 98.63,31.65 98.63,30.38 98.63,29.11 98.63,27.84 98.63,26.57 98.63,25.3 92.28,45.62 92.28,44.35 92.28,43.08 92.28,41.81 92.28,40.54 92.28,39.27 110.52,18.9 109.25,18.9 110.57,20.47 109.86,11.94 108.48,11.94 109.86,10.46 108.48,10.46 102.39,11.53 100.41,14.17 96.34,14.43 96.9,9.55 98.37,9.55 94.16,4.67 95.58,4.67 100.2,3.86 101.57,3.86 106.76,3.96 78.97,12.14 78.97,10.67 78.97,9.14 74.04,9.19 74.04,7.72 68.35,14.63 64.64,24.03 64.64,25.45 63.58,65.28 72.11,63.25 72.16,56.34 72.11,61.77 63.73,68.99 64.69,67.97 65.66,67.01 87.71,60.5 91.11,57.51 88.11,76.96 104.17,92.91 102.59,92.91 91.26,93.01 92.79,93.01 91.67,85.7 89.43,86.56 99.44,82.35 80.95,105.56 79.43,105.56 77.9,105.56 49.86,82.6 53.72,79.86 52.81,84.89 46,61.77 38.58,63.09 46,56.95 23.09,38.96 23.09,40.49 23.04,53.59 23.04,55.12 20.9,97.89 20.9,99.31 20.9,100.84 115.54,28.75 115.49,27.28 115.49,25.7 115.24,21.64 115.24,20.37 111.89,33.22 111.89,31.65 115.29,68.53 115.29,69.95 80.04,24.99 63.17,32.16 62.71,35.81 62.46,39.07 62.38,43.54 55.4,26.42
  pour Bottom (isolate 0.508): 26.29,124.21 26.29,110.24 23.75,107.7 23.75,16.26 -0.38,16.26 -0.38,124.21
  pour Bottom: 27.56,124.21 107.87,124.21 107.87,109.63 112.65,104.85 112.65,16.26 135.51,16.26 135.51,0.05 -0.18,0.05 -0.18,15.19 24.87,15.19 24.87,107.19 27.56,109.88
  pour Bottom (isolate 0.508): 135.51,124.21 109.35,124.16 109.35,109.88 113.87,105.21 113.61,17.12 135.56,17.12
  pour Top (isolate 0.508): -0.38,125.48 21.46,125.53 21.46,16.31 -1.65,16.26 -1.65,125.48
  pour Top (isolate 0.508): 113.92,125.48 113.92,16.26 135.51,16.26 135.51,125.48
  pour Top: 112.65,125.48 112.65,14.99 135.51,14.99 135.51,-0.25 -0.38,-0.25 -0.38,13.72 -0.38,14.99 22.48,14.99 22.48,125.48
  pour Bottom: 111.38,70.87 115.19,70.87 115.19,69.6 111.38,69.6
  pour Bottom: 111.38,48.01 115.19,48.01 115.19,49.28 111.38,49.28
  pour Bottom: 111.38,35.31 115.19,35.31 115.19,34.04 111.38,34.04
  pour Bottom: 111.38,20.07 115.19,20.07 115.19,21.34 111.38,21.34
HALL1
  Top 0.305: R53.1 89.68,81.48 R52.2
  Top 0.406: R53.1 89.68,84.57 88.01,86.23 88.01,99.69 90.04,101.73 U$17.46
HALL2
  Top 0.305: R54.2 105.52,81.61 R55.2
  Top 0.406: R54.2 105.52,84.57 109.09,88.14 109.09,99.77 111.63,102.31 111.63,115.03 U$17.39
HC1
  Top 0.305: LED17.C 121.39,26.13 R143.2 125.28,25.97 D27.A
  Top 1.676: U$3.D 122.64,22.69 D27.A
  Bottom 1.676: D27.A 127.51,25.65 131.32,29.46 131.32,104.65 126.49,109.47 126.49,112.01 123.44,115.06 123.44,116.64 U$17.42
HC1_CPU  (via drill 0.5)
  Top 0.305: IC2.9 106.43,49.91 v106.05,49.53
  Bottom 0.305: v106.05,49.53 105.54,49.02 99.44,49.02 98.55,49.91 84.07,49.91 80.8,46.63 80.8,40.54 77.98,37.72 77.98,27.94 | 77.98,27.94 U$1.6 | R6.2 78.94,26.97 77.98,27.94
HC1_TC4
  Top 0.305: U$3.G 113.22,23.23 | 113.22,23.23 R18.1 | 113.22,23.23 113.22,26.61 110.87,28.96 110.87,43.69 110.24,44.32 110.24,50.55 109.6,51.18 IC2.10
HC2
  Top 0.305: LED16.C 121.57,40.23 R141.2 125.41,40.33 D26.A
  Top 1.676: U$2.D 122.64,36.41 125.35,39.12 | 125.35,39.12 D26.A | 125.35,39.12 128.02,39.12 130.68,41.78 130.68,108.2 124.74,114.15 120.98,114.15 120.02,115.11 U$17.41
HC2_CPU  (via drill 0.5)
  Top 0.305: IC2.11 107.19,52.45 v104.9,50.16 | R7.2 75.03,27.79 U$1.7
  Bottom 0.305: v104.9,50.16 104.39,49.66 99.82,49.66 98.93,50.55 83.69,50.55 80.19,47.04 80.19,40.95 77.22,37.97 77.22,29.72 U$1.7
HC2_TC4
  Top 0.305: 115.34,37.21 U$2.G 113.34,37.46 | 113.34,37.46 R20.1 | 113.34,37.46 113.34,42.23 111,44.58 111,52.58 109.86,53.72 IC2.12
IAT  (via drill 0.5)
  Top 0.305: R40.2 14.54,6.8 | 14.54,6.8 D6.C 14.54,6.66 C10.1 | 14.54,6.8 16.57,6.8 D5.A 19.05,7.24 v19.68,7.87 | v39.5,15.62 R76.2
  Bottom 0.305: v19.68,7.87 23.19,7.87 30.96,15.65 39.47,15.65 v39.5,15.62
IAT_CPU  (via drill 0.5)
  Top 0.305: U3.2 U3.1 49.66,16.51 v50.42,15.75
  Bottom 0.305: U$1.A11 64.52,19.3 64.52,17.4 64.01,16.89 51.56,16.89 v50.42,15.75
IAT_SENSOR
  Top 0.254: 12.65,12.96 R41.1
  Top 0.305: R41.1 12.64,10.93 C9.1 12.63,8.89 R40.1
  Top 0.406: R41.1 10.92,13.97 3.43,21.46 3.43,51.94 1.91,53.47 1.91,105.66 10.41,114.17 10.41,117.6 12.06,119.25 26.92,119.25 28.45,117.73 28.45,116.91 U$17.6
IDLE
  Top 0.305: LED18.C 121.44,54.7 R145.2 125.16,54.8 D28.A
  Top 1.676: U$5.D 122.64,51.4 D28.A 126.87,54.36 128.02,55.5 128.02,102.49 123.83,106.68 121.92,106.68 120.14,108.46 120.14,111.81 U$17.55
IDLE_CPU  (via drill 0.5)
  Top 0.305: IC2.14 106.81,56.26 105.03,54.48 105.03,52.2 v104.65,51.82 | U$1.10/CS 75.18,35.94 74.55,35.31 73.5,35.31 R9.2
  Bottom 0.305: v104.65,51.82 83.19,51.82 78.92,47.55 78.92,41.61 77.06,39.75 74.93,39.75 74.3,39.12 74.3,37.47 U$1.10/CS
IDLE_TC4
  Top 0.305: U$5.G 113.09,51.94 R38.1 112.78,56.26 111.51,57.53 IC2.15
IGN1
  Top 0.406: R68.2 74.06,104.54 76.33,106.81 78.23,106.81 80.01,108.58 80.01,111.91 U$17.43
IGN1_CPU  (via drill 0.5)
  Top 0.254: U$9.2 77.6,93.5 77.19,93.09 75.36,93.09 75.06,92.79 75.06,91.81 R66.1
  Top 0.305: R66.1 75,90.74 75.69,90.04 75.69,89.22 R30.2 76.71,89.15 77.47,88.39 77.47,85.85 76.07,84.45 74.04,84.45 72.39,82.8 v72.39,73.15
  Bottom 0.305: U$1.29 75.82,59.18 77.98,61.34 77.98,70.99 75.18,73.79 73.03,73.79 v72.39,73.15
IGN2
  Top 0.406: R67.2 82.43,110.99 U$17.44
IGN2_CPU  (via drill 0.5)
  Top 0.254: U$9.4 80.14,93.7 80.54,93.29 81.15,93.29 81.46,92.99 81.46,91.81 R63.2
  Top 0.305: R63.2 81.52,90.79 80.77,90.04 80.77,89.21 R31.2 79.76,89.15 79.12,88.52 79.12,86.49 76.45,83.82 74.42,83.82 73.15,82.55 73.15,73.41 v74.04,72.52
  Bottom 0.305: U$1.30 76.45,61.34 77.34,62.23 77.34,70.74 75.56,72.52 v74.04,72.52
IGN3
  Top 0.406: R36.2 58.57,103.35 58.57,110.06 56.72,111.91 55.28,111.91 U$17.28
IGN3_CPU
  Top 0.254: R34.1 59.86,92.65 60.3,93.09 62.08,93.09 62.53,93.55 62.53,94.76 U$11.2
  Top 0.305: R34.1 59.86,91.14 60.58,90.42 60.58,89.22 R120.2 61.72,89.15 62.26,88.62 62.26,71.93 63.83,70.36 65.56,70.36 67.69,68.22 73.69,68.22 74.55,67.36 74.55,65.48 75.82,64.21 U$1.31/A12
IGN4
  Top 0.406: 67.34,104.37 R35.2 67.33,110.03 63.96,113.41 36.83,113.41 35.31,114.93 35.31,116.71 U$17.8
IGN4_CPU
  Top 0.254: U$11.4 65.02,93.55 65.28,93.29 65.89,93.29 66.29,92.89 66.29,91.71 R33.2
  Top 0.305: 66.29,91.71 66.29,90.93 65.53,90.17 65.53,89.09 R121.2 63.37,89.03 62.87,88.52 62.87,72.24 64.14,70.97 65.81,70.97 67.89,68.88 75.11,68.88 75.82,68.17 U$1.32/A13
IGN5
  Top 0.406: U$17.24 41.91,111.93 41.91,109.73 35.94,103.76 35.94,86.11 35.38,85.55 JP15.2
IGN5_CPU  (via drill 0.5)
  Top 0.254: R105.1 30.21,75.23 R112.2 30.26,75.15 30.79,74.62 32.66,74.62 33.68,73.61 33.68,72.15 U$25.2
  Top 0.305: 33.68,72.15 33.68,70.59 34.8,69.47 36.45,69.47 37.34,68.58 52.2,68.58 53.47,67.31 v53.47,66.42 | v62.05,62.69 62,62.69 61.95,62.64 v55.24,62.64
  Bottom 0.305: v53.47,66.42 53.34,66.29 53.34,63.5 54.2,62.64 v55.24,62.64 | U$1.28 75.82,56.74 74.55,58.01 74.55,59.44 73.84,60.15 63.83,60.15 62.2,61.77 62.2,62.54 v62.05,62.69
IGN6
  Top 0.406: U$17.25 45.21,111.9 45.21,110.11 38.35,103.25 38.35,85.06 JP18.1
IGN6_CPU  (via drill 0.5)
  Top 0.254: R104.2 R113.2
  Top 0.305: R113.2 38.52,75.18 37.34,75.18 36.2,74.04 U$25.4 36.2,70.74 37.72,69.21 52.83,69.21 v53.09,68.96 | 55.09,41.45 v55.07,41.48 55.04,41.45 55.04,40.13 56.69,38.48 U$1.14/A0
  Bottom 0.305: v53.09,68.96 51.82,67.69 51.82,53.72 53.01,52.53 53.01,47.65 54.48,46.18 54.48,42.06 v55.07,41.48
IGN7
  Top 0.406: U$17.26 48.64,111.9 48.64,108.2 47.24,106.81 43.94,106.81 40.89,103.76 40.89,87.25 41.27,86.87 42.49,86.87 42.95,86.41 42.95,84.89 JP16.2
IGN7_CPU  (via drill 0.5)
  Top 0.305: R109.1 48.04,77.6 R114.2 50.55,75.18 51.74,73.99 U$26.2 51.74,71.58 51.82,71.5 51.82,70.48 52.32,69.98 53.47,69.98 54.36,69.09 54.36,65.91 53.34,64.9 53.34,57.51 54.43,56.41 v54.91,56.41
  Bottom 0.305: U$1.39/A20 60.6,51.18 61.9,52.48 61.9,54.25 61.19,54.97 59.46,54.97 58.04,56.39 54.94,56.39 v54.91,56.41
IGN8
  Top 0.406: U$17.27 51.94,111.92 51.94,108.71 49.28,106.05 45.72,106.05 43.43,103.76 43.43,87.88 44.3,87.02 46.81,87.02 48.08,85.75 JP17.1
IGN8_CPU  (via drill 0.5)
  Top 0.254: R108.2 56.61,75.21 R115.2
  Top 0.305: R115.2 55.37,75.18 54.28,74.09 U$26.4 54.28,70.81 v55.37,69.72
  Bottom 0.305: U$1.22/A8 60.58,18.67 61.85,19.94 61.85,21.34 62.74,22.22 62.74,23.95 61.95,24.74 61.95,25.96 60.88,27.03 59.59,27.03 58.55,28.07 58.55,29.31 57.12,30.73 57.12,40.84 55.09,42.88 55.09,46.48 53.62,47.96 53.62,52.93 52.45,54.1 52.45,66.8 v55.37,69.72
INJ1_CPU  (via drill 0.5)
  Top 0.305: IC1.7 30.35,51.18 30.99,50.55 30.99,48.9 39.5,40.39 39.5,33.15 38.73,32.39 v38.73,32.26 | v71.53,30.2 71.22,29.84 63.55,29.84 62.05,31.34 62.05,34.04 61.42,34.67 56.95,34.67 54.53,32.26 v50.65,32.26 51.06,31.84 R12.2
  Bottom 0.305: v38.73,32.26 v50.65,32.26 | v71.53,30.2 71.35,29.97 71.35,30.07 71.65,30.38 71.65,32.66 72.36,33.38 75.79,33.38 U$1.9/CS
INJ1_TC4
  Top 0.305: U$12.G 22.93,18.42 R3.1 24.07,18.48 24.64,19.05 24.64,32.51 25.27,33.15 25.27,46.74 26.04,47.5 26.04,52.07 26.42,52.45 IC1.6
INJ2_CPU  (via drill 0.5)
  Top 0.305: IC1.5 30.48,53.72 31.62,52.58 31.62,49.15 40.02,40.75 40.13,40.64 40.16,40.62 40.16,31.75 38.28,29.87 38.28,25.91 34.16,21.79 34.16,8.28 34.8,7.64 v34.8,7.62 | R13.2 67.44,27.79 68.86,29.21 74.17,29.21 U$1.8
  Bottom 0.305: v34.8,7.62 35.05,7.62 35.69,6.98 57.15,6.98 58.93,5.21 76.15,5.21 77.9,6.96 77.9,23.27 76.68,24.49 74.95,24.49 74.42,25.02 74.42,29.46 U$1.8
INJ2_TC4
  Top 0.305: U$4.G 22.92,32.9 R5.1 24.07,32.83 24.64,33.4 24.64,46.99 25.4,47.75 25.4,54.36 25.91,54.86 28.17,54.86 IC1.4
INJ3_CPU  (via drill 0.5)
  Top 0.305: IC1.3 31.11,56.26 31.62,55.75 31.62,53.47 32.26,52.83 32.26,49.4 40.77,40.89 40.77,31.55 38.84,29.62 38.84,25.65 34.77,21.59 34.77,14.99 | v36.45,7.87 35.79,7.87 34.77,8.89 34.77,14.99 | R14.2 34.86,14.9 34.77,14.99
  Bottom 0.305: v36.45,7.87 36.45,7.75 36.58,7.62 57.4,7.62 59.18,5.84 75.82,5.84 77.29,7.31 77.29,21.77 U$1.5
INJ3_TC4
  Top 0.305: U$6.G 22.93,47.38 R8.1 24.2,47.44 24.77,48.01 24.77,56.77 25.53,57.53 IC1.2
INJ4_CPU  (via drill 0.5)
  Top 0.305: IC1.9 36.07,49.91 36.58,49.4 36.58,45.85 41.4,41.02 41.4,27.18 | v56.01,15.88 56.01,16.26 53.72,18.54 47.37,18.54 45.21,20.7 45.21,23.37 41.4,27.18 | v64.95,12.37 64.95,12.29 72.92,12.29 75.41,14.78 75.41,15.21 U$1.2 | R15.2 37.41,23.19 41.4,27.18
  Bottom 0.305: v56.01,15.88 56.01,15.11 59.31,11.81 64.39,11.81 v64.95,12.37
INJ4_TC4
  Top 0.305: U$8.G 22.93,62.11 R11.1 27.62,62.17 30.86,58.93 30.86,57.66 32.13,56.39 32.13,53.85 32.89,53.09 32.89,51.56 33.27,51.18 IC1.10
INJ5_CPU
  Top 0.305: IC1.11 36.45,52.45 37.21,51.69 37.21,46.1 39.62,43.69 44.07,43.69 45.59,42.16 53.31,42.16 54.08,41.4 54.08,40.18 57.07,37.19 62.2,37.19 65.25,40.23 72.77,40.23 | 72.77,40.23 75.03,40.23 U$1.12/MISO | R16.2 73.06,40.25 72.77,40.23
INJ5_TC4
  Top 0.305: U$19.G 20.29,74.43 R88.1 20.28,74.42 21.08,74.42 21.97,73.53 21.97,68.83 31.5,59.31 31.5,57.91 32.77,56.64 32.77,54.1 33.15,53.72 IC1.12
INJ6_CPU
  Top 0.305: IC1.14 36.7,56.26 37.85,55.12 37.85,46.36 39.9,44.3 44.37,44.3 45.9,42.77 47.88,42.77 | U$1.27 77.34,52.2 77.34,50.67 76.58,49.91 75.18,49.91 74.42,49.15 74.42,45.44 73.53,44.55 70.89,44.55 68.5,42.16 65.35,42.16 64.44,41.25 62.66,41.25 61.14,39.73 56.82,39.73 56.01,40.54 56.01,41.86 55.09,42.77 47.88,42.77 | R10.2 47.84,42.81 47.88,42.77
INJ6_TC4
  Top 0.305: IC1.15 32.77,57.53 32.13,58.17 32.13,59.69 22.73,69.09 22.73,73.91 21.84,74.8 21.84,88.65 21.08,89.41 20.39,89.41 R89.1 20.29,89.32 U$20.G
INJ7_CPU  (via drill 0.5)
  Top 0.305: IC2.3 100.08,56.26 v99.95,56.13
  Bottom 0.305: v99.95,56.13 99.19,55.37 99.19,53.72 98.55,53.09 82.68,53.09 79.38,49.78 75.06,49.78 | 75.06,49.78 74.17,48.9 74.17,47.75 U$1.24 | R1.2 73.69,51.16 75.06,49.78
INJ7_TC4
  Top 0.305: U$21.G 112.78,96.26 R90.1 111.49,95.87 110.49,94.87 110.49,80.77 109.73,80.01 109.73,66.29 107.95,64.52 105.03,64.52 103.76,63.25 103.76,57.91 103.38,57.53 IC2.2
INJ8_CPU  (via drill 0.5)
  Top 0.305: IC2.5 v100.08,53.72
  Bottom 0.305: v100.08,53.72 98.81,52.45 82.93,52.45 79.12,48.64 | 79.12,48.64 U$1.25 | R2.2 72.81,41.18 73.94,42.32 77.75,42.32 78.31,42.88 78.31,47.83 79.12,48.64
INJ8_TC4
  Top 0.305: U$22.G 112.94,81.27 | 112.94,81.27 R91.1 | 112.94,81.27 112.01,81.27 110.36,79.63 110.36,65.91 108.25,63.8 105.28,63.8 104.52,63.04 104.52,56.01 103.5,54.99 IC2.4
INJECTOR1
  Top 0.254: 10.1,25.72 10.03,25.72 D22.A
  Top 0.305: 10.1,25.72 R103.2 17.68,25.72 LED12.C | U$12.D 12.99,22.52 13.59,23.11
  Top 1.676: U$12.D 12.99,22.69 D22.A
  Bottom 1.676: U$17.1 11.96,115.59 9.14,112.78 9.14,111.12 4.57,106.55 4.57,27.69 6.54,25.72 10.03,25.72 D22.A
INJECTOR2
  Top 0.305: D23.A 10.22,40.2 R134.2 13.69,40.1 LED13.C | U$4.D 12.99,36.36 13.59,36.96
  Top 1.676: U$4.D 12.99,37.43 D23.A 7.24,40.26 6.35,41.15 6.35,52.83 4.7,54.48 4.7,104.52 9.27,109.09 11.3,109.09 11.94,109.73 11.94,111.92 U$17.15
INJECTOR3
  Top 0.305: D24.A 10.47,54.68 R136.2 13.74,54.83 LED14.C | U$6.D 12.99,51.22 13.59,51.82
  Top 1.676: U$6.D 12.99,52.16 D24.A 8,54.86 7.37,55.5 7.37,103.38 10.29,106.3 13.46,106.3 15.37,108.2 15.37,111.87 U$17.16
INJECTOR4
  Top 0.305: D25.A 10.35,69.41 R139.2 13.74,69.56 LED15.C | U$8.D 12.99,66.08 13.59,66.67
  Top 1.676: 12.99,66.08 12.99,66.63 D25.A
  Bottom 1.676: D25.A 18.01,69.34 23.09,74.42 23.09,109.76 U$17.19
INJECTOR5
  Top 0.305: U$19.D 12.99,80.68 13.59,81.28 | D4.A 10.35,84.14 R81.2 17.63,84.14 LED8.C
  Top 1.676: U$19.D 12.99,81.37 D4.A
  Bottom 1.676: U$17.18 18.82,108.82 18.82,88.29 14.61,84.07 D4.A
INJECTOR6
  Top 0.305: LED9.C 13.69,98.77 R85.2 10.61,98.87 D14.A | U$20.D 12.99,95.29 13.59,95.88
  Top 1.676: U$20.D 12.99,95.84 D14.A 17.91,98.55 18.62,99.26 U$17.17 18.67,111.9
INJECTOR7
  Top 0.305: LED10.C 121.44,99.03 R87.2 125.03,99.13 D20.A
  Top 1.676: U$21.D 122.13,95.59 D20.A 116.2,98.81 115.06,99.95 115.06,107.31 116.71,108.97 116.71,111.91 U$17.54
INJECTOR8
  Top 0.305: LED11.C 121.51,83.91 R101.2 125.03,83.89 D21.A
  Top 1.676: U$22.D 122.13,80.35 D21.A
  Bottom 1.676: D21.A 119.38,83.57 117.22,85.72 117.22,107.06 113.67,110.62 113.67,111.63 U$17.53
LC1
  Top 0.406: Q3.3 39.8,46.81 38.61,48.01 38.61,58.8 34.8,62.61 30.35,62.61 23.5,69.47 23.5,74.3 22.61,75.18 22.61,107.44 20.57,109.47 20.57,112.39 19.56,113.41 16.51,113.41 15.37,114.55 15.37,116.67 U$17.2
LC1_CPU  (via drill 0.5)
  Top 0.305: v52.7,45.85 52.7,47.04 51.38,48.36 49.82,48.36 R62.2
  Bottom 0.305: U$1.20/A6 59.94,23.24 57.28,25.91 57.28,28.7 55.8,30.17 55.8,38.46 53.21,41.05 53.21,44.91 52.7,45.41 v52.7,45.85
MAP_CONV
  Top 0.305: R124.2 97.69,19.94 100.33,17.3 JP20.1
MAP_CPU
  Top 0.305: U2.8 U2.9 | U2.9 80.26,14.99 | U$1.17/A3 59.18,29.46 59.18,25.15 59.82,24.51 61.34,24.51 64.34,21.51 64.34,20.01 65.91,18.44 65.91,14.73 63.88,12.7 63.88,11.68 64.34,11.23 74.5,11.23 75.06,11.79 76.58,11.79 79.73,14.94 80.59,14.94 U2.9
MAP_EXT
  Top 0.406: U$17.49 100.03,106.95 JP22.1
MISO2
  Top 0.305: JP7.1 64.41,52.43 U$1.51
MOSI2
  Top 0.305: JP6.1 57.33,49.89 57.43,49.99 57.43,49.89 62.36,49.89 63.58,48.67 65.63,48.67 U$1.52
N$1
  Top 0.305: R80.2 17.02,88.65 17.78,87.88 LED8.A
N$2
  Top 0.305: R82.2 118.75,73.79 117.98,73.02 LED5.A
N$3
